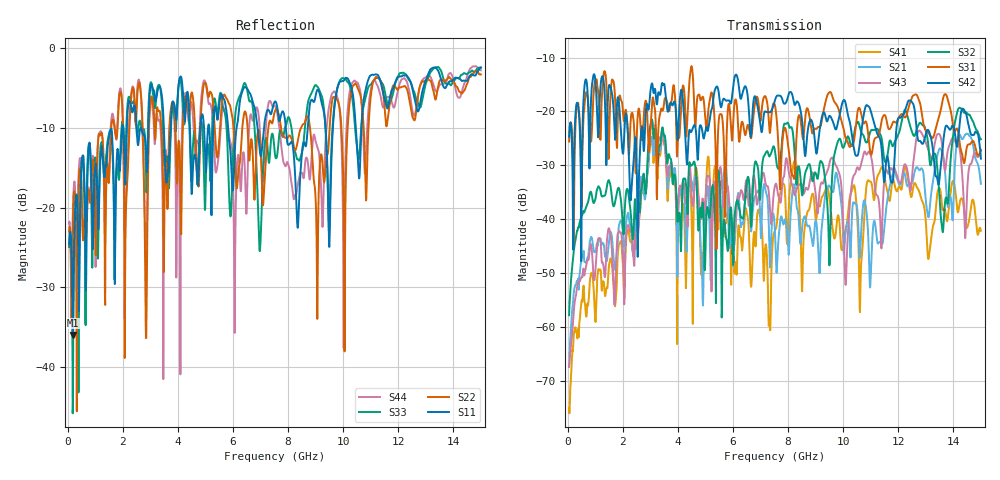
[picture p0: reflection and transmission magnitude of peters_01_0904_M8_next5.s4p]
# MHZ S RI R 50.00
! FREQ  S11  S12  S13  S14
!  S21  S22  S23  S24
!  S31  S32  S33  S34
!  S41  S42  S43  S44
!  REAL  IMAG  REAL  IMAG  REAL  IMAG  REAL  IMAG
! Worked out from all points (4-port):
!   1496 points, 50 MHz to 15 GHz, reference 50 ohm
!   strongest paths, dB at 50 MHz, 3.79 GHz, 7.53 GHz, 11.27 GHz, 15 GHz:
!     S42: -24.7, -18.8, -17.8, -24.5, -28.8
!     S31: -25.6, -17.3, -19.0, -24.6, -27.1
!     S32: -57.8, -31.9, -27.6, -23.5, -25.2
!     S43: -67.4, -30.5, -33.7, -35.9, -27.3
!     S21: -67.4, -30.9, -43.1, -44.5, -33.4
!     S41: -75.0, -31.0, -42.0, -31.7, -42.1
!   lowest |S11| = -36.0 dB at 190 MHz (marker M1), VSWR 1.03, Z = 48.8 + j1.02 ohm
!   |S11| at or under -10 dB: start of sweep to 1.977 GHz; 4.437 GHz to 4.813 GHz (376.7 MHz wide, 8.15 % of centre); 7.919 GHz to 8.712 GHz (793.2 MHz wide, 9.54 % of centre)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
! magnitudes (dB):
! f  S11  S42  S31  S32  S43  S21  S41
! 50 MHz  -24.6  -24.7  -25.6  -57.8  -67.4  -67.4  -75.0
! 190 MHz  -36.0  -41.9  -29.4  -47.3  -59.3  -55.3  -63.9
! 3.46 GHz  -7.8  -15.1  -19.7  -23.5  -23.7  -24.9  -24.7
! 5.64 GHz  -6.3  -17.8  -22.9  -41.6  -37.5  -34.0  -36.2
! 7.32 GHz  -7.9  -20.1  -23.3  -28.4  -36.2  -45.7  -58.4
! 8.25 GHz  -15.6  -18.8  -31.3  -28.7  -35.5  -34.2  -29.2
! 15 GHz  -2.4  -28.8  -27.1  -25.2  -27.3  -33.4  -42.1
